TYPE dut_PLC_to_PMC :
STRUCT
	bHeartBeatMonitor	: BOOL;		

	//interlock status
	DP					,
	BWR					,
	DPR1				,
	DPR2				,
	WAT_R				,
	WAT_F				,
	HTR1				,
	HTR2				,
	HTR3				,
	HTR4				,
	HTR5				,
	T_MNT				,
	T_REF				,
	DEPO				,
	CLN					,
	ECO					,
	AGV					,
	SP1					,
	PZ					,
	P_CONT				,
	DGZERO				,
	C_EXH				,
	F2_CLN				,
	F_N					
	: BOOL;
	
	//automatic valve status
	P_RUN				,
	LSC1_Level_HH		,
	LSC1_Level_H		,
	LSC1_Level_M		,
	LSC1_Level_L		,
	LSC1_OverFill		,
	LSC1_Ref_RDY		,
	T_REF_On			,
	D_Gas_OK			,
	DEPO_OK				,
	CLN_OK				,
	ATM					,
	F2_CLN_OK			,
	VAC1				,
	VAC2				,
	VAC3				,
	VAC4				,
	VAC5				
	: BOOL;
	

	aILK_AV				: ARRAY[1..250]	OF BOOL;
	aVAC				: ARRAY[1..10]	OF BOOL;
	bAV540				: BOOL;
	bBoatUnLoad_ILK		: BOOL;// boat unload condition
	stIntlk				: dut_Interlock ;
	
	
	//Gas box input
	
	I200_00			:BOOL;	//	PG3_LOW_ALARM
	I200_01			:BOOL;	//	PG3_HIGH_ALARM
	I200_02			:BOOL;	//	PG4_LOW_ALARM
	I200_03			:BOOL;	//	PG4_HIGH_ALARM
	I200_04			:BOOL;	//	PG5_LOW_ALARM
	I200_05			:BOOL;	//	PG5_HIGH_ALARM
	I200_06			:BOOL;	//	PG6_LOW_ALARM
	I200_07			:BOOL;	//	PG6_HIGH_ALARM
	I200_08			:BOOL;	//	PG7_LOW_ALARM
	I200_09			:BOOL;	//	PG7_HIGH_ALARM
	I200_10			:BOOL;	//	PG8_LOW_ALARM
	I200_11			:BOOL;	//	PG8_HIGH_ALARM
	I200_12			:BOOL;	//	PG31_LOW_ALARM
	I200_13			:BOOL;	//	PG31_HIGH_ALARM
	I200_14			:BOOL;	//	PG32_LOW_ALARM
	I200_15			:BOOL;	//	PG32_HIGH_ALARM
	I201_00			:BOOL;	//	LSC_H_LEVEL
	I201_01			:BOOL;	//	LSC_M_LEVEL
	I201_02			:BOOL;	//	LSC_L_LEVEL
	I201_03			:BOOL;	//	VG31_STATUS_OK
	I201_04			:BOOL;	//	VG31_LOW_ALARM
	I201_05			:BOOL;	//	VG31_HIGH_ALARM
	I201_06			:BOOL;	//	GD_FAN1_STOP
	I201_07			:BOOL;	//	GD_FAN2_STOP
	I201_08			:BOOL;	//	OX_MS1
	I201_09			:BOOL;	//	OX_MS2
	I201_10			:BOOL;	//	OX_MS3
	I201_11			:BOOL;	//	OX_MSI1
	I201_12			:BOOL;	//	OX_MSI2
	I201_13			:BOOL;	//	OX_RC1
	I201_14			:BOOL;	//	OX_RC2
	I201_15			:BOOL;	//	OX_RC3
	I202_00			:BOOL;	//	MS2_Pressure_LOW_ALARM
	I202_01			:BOOL;	//	MS2_Pressure_HIGH_ALARM
	I202_02			:BOOL;	//	MS321_Pressure_LOW_ALARM
	I202_03			:BOOL;	//	MS321_Pressure_HIGH_ALARM
	I202_04			:BOOL;	//	SPARE
	I202_05			:BOOL;	//	SPARE
	I202_06			:BOOL;	//	MP/PS20_Pressure_ALARM
	I202_07			:BOOL;	//	MP/PS11_Pressure_ALARM
	I202_08			:BOOL;	//	SPARE
	I202_09			:BOOL;	//	SPARE
	I202_10			:BOOL;	//	SPARE
	I202_11			:BOOL;	//	PG1_LOW_ALARM
	I202_12			:BOOL;	//	PG1_HIGH_ALARM
	I202_13			:BOOL;	//	PG2_LOW_ALARM
	I202_14			:BOOL;	//	PG2_HIGH_ALARM
	I202_15			:BOOL;	//	SPARE
	
	//Exhaust box input
	
	I300_00			:BOOL;	//	FS105_RHC_Flow_Alarm
	I300_01			:BOOL;	//	FS106_Heater_Jacket_Flow_Alarm
	I300_02			:BOOL;	//	FS202_Heater_Upper_Alarm
	I300_03			:BOOL;	//	FS104_Shutter_Flow_Alarm
	I300_04			:BOOL;	//	FS111_BoatRotation_Flow_Alarm
	I300_05			:BOOL;	//	FS102_Flange_Flow_Alarm
	I300_06			:BOOL;	//	Spare
	I300_07			:BOOL;	//	Spare
	I300_08			:BOOL;	//	VG11_Status_OK
	I300_09			:BOOL;	//	VG11_Low_Alarm
	I300_10			:BOOL;	//	VG11_High_Alarm
	I300_11			:BOOL;	//	VG13_Status_OK
	I300_12			:BOOL;	//	VG13_Low_Alarm
	I300_13			:BOOL;	//	VG13_High_Alarm
	I300_14			:BOOL;	//	AV71_Fan1_Alarm
	I300_15			:BOOL;	//	AV71_Fan2_Alarm
	I301_00			:BOOL;	//	DG1_Low_Limit_Alarm
	I301_01			:BOOL;	//	DG1_High_Limit_Alarm
	I301_02			:BOOL;	//	Spare
	I301_03			:BOOL;	//	Spare
	I301_04			:BOOL;	//	Spare
	I301_05			:BOOL;	//	Spare
	I301_06			:BOOL;	//	Spare
	I301_07			:BOOL;	//	Spare
	I301_08			:BOOL;	//	MP21/PS_Pressure_Low_Alarm
	I301_09			:BOOL;	//	FS101_MainWater_Flow_Alarm-1
	I301_10			:BOOL;	//	FS101_FMainWater_low_Alarm-2
	I301_11			:BOOL;	//	FL301_Flow_Switch
	I301_12			:BOOL;	//	FL72_Flow_Switch
	I301_13			:BOOL;	//	FS116_Zaxis_Flow_Alarm
	I301_14			:BOOL;	//	PS110_Pressure_Low_Alarm
	I301_15			:BOOL;	//	PS110_Pressure_High_Alarm
	I302_00			:BOOL;	//	PG/PS12_Pressure_Low_Alarm
	I302_01			:BOOL;	//	PG/PS12_Pressure_High_Alarm
	I302_02			:BOOL;	//	PS13_ATM_Status
	I302_03			:BOOL;	//	PS13_High_Limit_Alarm
	I302_04			:BOOL;	//	PG101_Water_Pressure_Low_Alarm
	I302_05			:BOOL;	//	PG101_Water_Pressure_High_Alarm
	I302_06			:BOOL;	//	VG14_Status_OK
	I302_07			:BOOL;	//	VG14_LOW_Alarm
	I302_08			:BOOL;	//	VG14_High_Alarm
	I302_09			:BOOL;	//	PS14_Pressure_Low_Alarm
	I302_10			:BOOL;	//	PS14_Pressure_High_Alarm
	I302_11			:BOOL;	//	Spare
	I302_12			:BOOL;	//	Spare
	I302_13			:BOOL;	//	Spare
	I302_14			:BOOL;	//	Spare
	I302_15			:BOOL;	//	Spare
	I303_00			:BOOL;	//	APC_Valve_Status
	I303_01			:BOOL;	//	APC_Alarm_Status
	I303_02			:BOOL;	//	RHC_Cooling_Air_cylinder1_Open
	I303_03			:BOOL;	//	RHC_Cooling_Air_cylinder1_Close
	I303_04			:BOOL;	//	RHC_Cooling_Air_cylinder2_Open
	I303_05			:BOOL;	//	RHC_Cooling_Air_cylinder2_Close
	I303_06			:BOOL;	//	RHC_Cooling_Valve_Open
	I303_07			:BOOL;	//	RHC_Cooling_Valve_Close
	I303_08			:BOOL;	//	RHC_Cooling_ButterflyValves_Open
	I303_09			:BOOL;	//	RHC_Cooling_ButterflyValves_Close
	I303_10			:BOOL;	//	Spare
	I303_11			:BOOL;	//	Spare
	I303_12			:BOOL;	//	GV_Open_NC
	I303_13			:BOOL;	//	GV_Open_NO
	I303_14			:BOOL;	//	GV_Close_NC
	I303_15			:BOOL;	//	GV_Close_NO
	I304_00			:BOOL;	//	RHC_Cooling_BallValve_Open
	I304_01			:BOOL;	//	RHC_Cooling_BallValve_Close
	I304_02			:BOOL;	//	Spare
	I304_03			:BOOL;	//	Spare
	I304_04			:BOOL;	//	Spare
	I304_05			:BOOL;	//	Spare
	I304_06			:BOOL;	//	Spare
	I304_07			:BOOL;	//	Spare
	I304_08			:BOOL;	//	Spare
	I304_09			:BOOL;	//	Spare
	I304_10			:BOOL;	//	Spare
	I304_11			:BOOL;	//	Spare
	I304_12			:BOOL;	//	Spare
	I304_13			:BOOL;	//	Spare
	I304_14			:BOOL;	//	Spare
	I304_15			:BOOL;	//	Spare	
	
	//Operation box input
	
	I600_00			:BOOL;	//	MS8_HC_ExhPress_LOW_ALARM
	I600_01			:BOOL;	//	MS8_HC_ExhPress_HIGH_ALARM
	I600_02			:BOOL;	//	MS1_Heater_ExhPress_LOW_ALARM
	I600_03			:BOOL;	//	MS1_Heater_ExhPress_HIGH_ALARM
	I600_04			:BOOL;	//	MS3_Scavenger_ExhPress_LOW_ALARM
	I600_05			:BOOL;	//	MS3_Scavenger_ExhPress_HIGH_ALARM
	I600_06			:BOOL;	//	MS6_Frontbody_ExhPress_LOW_ALARM
	I600_07			:BOOL;	//	MS6_Frontbody_ExhPress_HIGH_ALARM
	I600_08			:BOOL;	//	MS9_LSC1_ExhPress_LOW_ALARM
	I600_09			:BOOL;	//	MS9_LSC1_ExhPress_HIGH_ALARM
	I600_10			:BOOL;	//	MS11_GasBox_ExhPress_LOW_ALARM
	I600_11			:BOOL;	//	MS11_GasBox_ExhPress_HIGH_ALARM
	I600_12			:BOOL;	//	MS12_GasBox_ExhPress_LOW_ALARM
	I600_13			:BOOL;	//	MS12_GasBox_ExhPress_HIGH_ALARM
	I600_14			:BOOL;	//	SPARE
	I600_15			:BOOL;	//	SPARE
	
	//Sensor reading value
	
	PG3_Pressure		,	// IW250
	PG4_Pressure		,	// IW251
	PG5_Pressure		,	// IW252
	PG6_Pressure		,	// IW253
	PG7_Pressure		,	// IW254
	PG8_Pressure		,	// IW255
	PG31_Pressure		,	// IW256
	PG32_Pressure		,	// IW257
	VG31_Pressure		,	// IW258
	PG2_Pressure		,	// IW259
	PS11_Pressure		,	// IW260
	PG1_Pressure		,	// IW261
	MS2_Gasboxleft		,	// IW262
	MS5_Loadingarea		,	// IW263
	OX_Value			,	// IW264
                   	
	PG21_Pressure		,	// IW266
	PG22_Pressure		,	// IW267
	PG23_Pressure		,	// IW268
	PS33_Pressure		,	// IW269
	

	FS105_Flow			,	// IW300
	FS106_Flow          ,   // IW301
	FS202_Flow          ,   // IW302
	FS104_Flow          ,   // IW303
	FS111_Flow          ,   // IW304
	FS102_Flow          ,   // IW305
	DG1_Pressure        ,   // IW308
	FS116_Flow          ,   // IW311
	PS13_Pressure       ,   // IW312
	PS21_Pressure    	,   // IW318
	PS110_Pressure      ,   // IW319
	PG12_Pressure    	,   // IW320
	VG14_Pressure       ,   // IW321
	PS14_Pressure       ,   // IW322
	MS8_RHC_ExhPress    ,  	// IW332
	
	
	(*MS8_RHC_ExhPress		// IW600*)
	MS1_Heater			,	// IW601
	MS3_Scavenger		,	// IW602
	MS6_Frontbody		,	// IW603
	MS9_LSC1			,	// IW604
	MS11_GasBox			,	// IW605
	MS12_GasBox				// IW606
	:REAL;
	
	//FFU
	FFU1_1_STATUS	:	REAL	;	//	FFU1_1运行状态	
	FFU1_2_STATUS	:	REAL	;	//	FFU1_2运行状态	
	FFU1_3_STATUS	:	REAL	;	//	FFU1_3运行状态	
	FFU1_4_STATUS	:	REAL	;	//	FFU1_4运行状态	
	FFU1_5_STATUS	:	REAL	;	//	FFU1_5运行状态	
	FFU1_6_STATUS	:	REAL	;	//	FFU1_6运行状态	
	FFU2_1_STATUS	:	REAL	;	//	FFU2_1运行状态	
	FFU2_2_STATUS	:	REAL	;	//	FFU2_2运行状态	
	FFU2_3_STATUS	:	REAL	;	//	FFU2_3运行状态	
	FFU2_4_STATUS	:	REAL	;	//	FFU2_4运行状态	
	FFU2_5_STATUS	:	REAL	;	//	FFU2_5运行状态	
	FFU2_6_STATUS	:	REAL	;	//	FFU2_6运行状态	
	FFU3_1_STATUS	:	REAL	;	//	FFU3_1运行状态	
	FFU3_2_STATUS	:	REAL	;	//	FFU3_2运行状态	
	FFU3_3_STATUS	:	REAL	;	//	FFU3_3运行状态	
	FFU3_4_STATUS	:	REAL	;	//	FFU3_4运行状态	
	FFU3_5_STATUS	:	REAL	;	//	FFU3_5运行状态	
	FFU3_6_STATUS	:	REAL	;	//	FFU3_6运行状态	
		
	FFU1_1_SPEED_PV	:	REAL	;	//	FFU1_1当前转速	
	FFU1_2_SPEED_PV	:	REAL	;	//	FFU1_2当前转速	
	FFU1_3_SPEED_PV	:	REAL	;	//	FFU1_3当前转速	
	FFU1_4_SPEED_PV	:	REAL	;	//	FFU1_4当前转速	
	FFU1_5_SPEED_PV	:	REAL	;	//	FFU1_5当前转速	
	FFU1_6_SPEED_PV	:	REAL	;	//	FFU1_6当前转速	
	FFU2_1_SPEED_PV	:	REAL	;	//	FFU2_1当前转速	
	FFU2_2_SPEED_PV	:	REAL	;	//	FFU2_2当前转速	
	FFU2_3_SPEED_PV	:	REAL	;	//	FFU2_3当前转速	
	FFU2_4_SPEED_PV	:	REAL	;	//	FFU2_4当前转速	
	FFU2_5_SPEED_PV	:	REAL	;	//	FFU2_5当前转速	
	FFU2_6_SPEED_PV	:	REAL	;	//	FFU2_6当前转速	
	FFU3_1_SPEED_PV	:	REAL	;	//	FFU3_1当前转速	
	FFU3_2_SPEED_PV	:	REAL	;	//	FFU3_2当前转速	
	FFU3_3_SPEED_PV	:	REAL	;	//	FFU3_3当前转速	
	FFU3_4_SPEED_PV	:	REAL	;	//	FFU3_4当前转速	
	FFU3_5_SPEED_PV	:	REAL	;	//	FFU3_5当前转速	
	FFU3_6_SPEED_PV	:	REAL	;	//	FFU3_6当前转速	
	
	
END_STRUCT
END_TYPE
